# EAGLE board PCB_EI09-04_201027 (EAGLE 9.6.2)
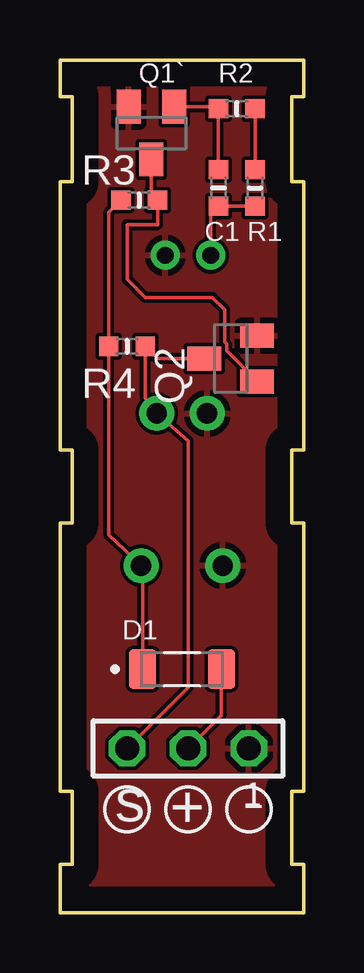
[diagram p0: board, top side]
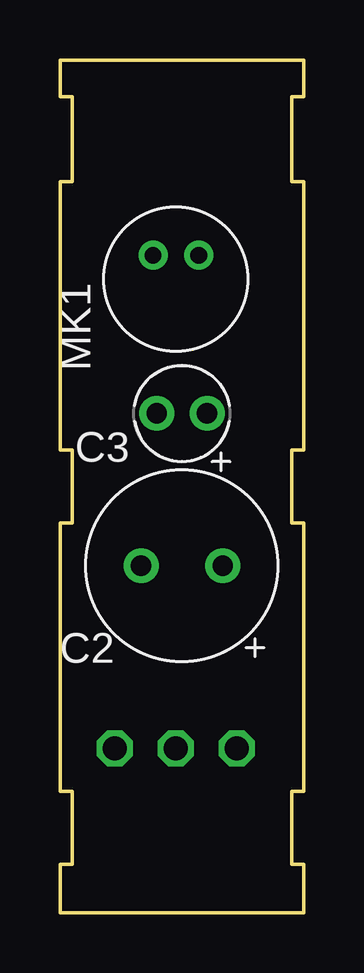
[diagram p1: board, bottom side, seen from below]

Size 10.16 x 35.56 mm. Coordinates in mm from the lower left corner, seen from the top.
Outline: 0,0 10.16,0 10.16,2.03 9.65,2.03 9.65,5.08 10.16,5.08 10.16,16.26 9.65,16.26 9.65,19.3 10.16,19.3 10.16,30.48 9.65,30.48 9.65,34.04 10.16,34.04 10.16,35.56 0,35.56 0,34.04 0.51,34.04 0.51,30.48 0,30.48 0,19.3 0.51,19.3 0.51,16.26 0,16.26 0,5.08 0.51,5.08 0.51,2.03 0,2.03 0,0
Copper layers (1*16): Top 0.035mm / dielectric 1.5mm / Bottom 0.035mm
Design rules "default": minimum track width 6mil, minimum drill 0.35mm, track to track 6mil, track to pad 6mil, pad to pad 6mil, via to via 6mil, smd to smd 6mil, copper to edge 40mil, drill to drill 6mil, minimum pad ring 10mil, minimum via ring 8mil, stop-mask expansion 4mil, vias tented up to drill 0mil, thermal gap 10mil

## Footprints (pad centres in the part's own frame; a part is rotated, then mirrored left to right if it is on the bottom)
RC-MASTER-SMD_C0603MP = smd 0.8 x 0.8: 1 -0.762,0; 2 0.762,0
CAPPRD340W65D800H550B = drill 0.85 pad 1.45: 1 -1.7,0; 2 1.7,0
CAPPRD210W65D400H540B = drill 0.85 pad 1.45: 1 -1.05,0; 2 1.05,0
DIOMELF3414N = smd 1.14 x 1.63: A 1.64,0; C -1.64,0
CUI_CMC-5042PF-AC = drill 0.7: GND 1,0.95; OUT 1,-0.95
SOT23-BEC = smd 1 x 1.4: B -0.95,-1.1; C 0,1.1; E 0.95,-1.1
RC-MASTER-SMD_R0603MP = smd 0.8 x 0.8: 1 -0.762,0; 2 0.762,0
TSW-103-XX-G-S = drill 1 pad 1.5 octagon: 1 2.54,0; 2 0,0; 3 -2.54,0

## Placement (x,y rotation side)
C1  1uF  [RC-MASTER-SMD_C0603MP]  6.6,30.23 270 top
C2  470uF  [CAPPRD340W65D800H550B]  5.08,14.48 180 bottom
C3  100uF  [CAPPRD210W65D400H540B]  5.08,20.83 180 bottom
D1  FDLL4148  [DIOMELF3414N]  5.08,10.16 0 top
MK1  CMC-5042PF-AC  [CUI_CMC-5042PF-AC]  5.33,26.42 90 bottom
Q1`  MMBT2222ALT1  [SOT23-BEC]  3.81,32.51 180 top
Q2  MMBT2222ALT1  [SOT23-BEC]  7.11,23.11 90 top
R1  2K  [RC-MASTER-SMD_R0603MP]  8.13,30.23 90 top
R2  910K  [RC-MASTER-SMD_R0603MP]  7.37,33.53 180 top
R3  10K  [RC-MASTER-SMD_R0603MP]  3.3,29.72 0 top
R4  4.7K  [RC-MASTER-SMD_R0603MP]  2.79,23.62 0 top
X1  TSW-103-07-G-S  [TSW-103-XX-G-S]  5.33,6.86 0 top

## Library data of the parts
C1 R1-R4 = 52101-101-REV-A_v16
C2 C3 = EI09-04
D1 = FDLL4148; DESCRIPTION: Diode Standard 100V 200mA Surface Mount SOD-80; DIGI-KEY_PART_NUMBER: FDLL4148CT-ND; MF: ON Semiconductor; MP: FDLL4148; PACKAGE: SOD-80-2 ON Semiconductor; PURCHASE-URL: https://pricing.snapeda.com/search/part/FDLL4148/?ref=eda
MK1 = CMC-5042PF-AC; AVAILABILITY: Good; CUI_PURCHASE_URL: https://www.cuidevices.com/product/audio/microphones/electret-condenser-microphones/cmc-5042pf-ac?utm_source=snapeda.com&utm_medium=referral&utm_campaign=snapedaBOM; DESCRIPTION: 6.0 mm, Omnidirectional, PCB Mount, 2.0 Vdc, Electret Condenser Microphone; MF: CUI Devices; MP: CMC-5042PF-AC; PACKAGE: CUI Inc.; PRICE: None; PURCHASE-URL: https://pricing.snapeda.com/search/part/CMC-5042PF-AC/?ref=eda
Q1` Q2 = transistor-neu-to92
X1 = con-samtec; MF: Samtec Inc.; MPN: TSW-103-07-G-S

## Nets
GND: C2.2 C3.2 MK1.OUT Q1`.E Q2.E X1.1
N$1: D1.A X1.2
N$2: C3.1 Q2.C R4.2 X1.3
N$3: C1.1 Q1`.B R2.2
N$4: R1.2 R2.1
N$5: C1.2 MK1.GND R1.1
N$6: Q1`.C Q2.B R3.2
N$7: C2.1 D1.C R3.1 R4.1

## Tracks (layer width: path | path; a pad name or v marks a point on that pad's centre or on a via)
GND
  pour Top: 0,35.56 10.16,35.56 10.16,0 0,0
N$1
  Top 0.152: X1.2 6.72,8.24 D1.A
N$2
  Top 0.152: X1.3 5.33,9.4 5.33,19.68 C3.1 3.56,21.46 R4.2 4.06,23.11 Q2.C
N$3
  Top 0.152: Q1`.B 6.52,33.61 R2.2 C1.1
N$4
  Top 0.152: R2.1 R1.2
N$5
  Top 0.152: C1.2 R1.1 | 6.6,29.14 C1.2 | MK1.GND 6.28,29.14 C1.2
N$6
  Top 0.152: Q1`.C 3.81,29.97 R3.2 4.06,28.7 2.79,28.7 2.79,26.42 3.56,25.65 6.35,25.65 6.86,25.15 6.86,23.79 6.94,23.71 6.94,23.43 Q2.B
N$7
  Top 0.152: D1.C 3.44,14.34 C2.1 2.03,15.75 R4.1 2.03,29.21 R3.1

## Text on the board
tPlace: s | + | -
